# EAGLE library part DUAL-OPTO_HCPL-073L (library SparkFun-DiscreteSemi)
HCPL-073L These high gain series couplers use a Light Emitting Diode and an integrated high gain photodetector to provide extremely high current transfer ratio between input and output. Separate pins for the photodiode and output stage result in LVTTL compatible saturation voltages and high speed operation. Where desired, the VCC and VO terminals may be tied together to achieve conventional photo-darlington operation. A base access terminal allows a gain bandwidth adjustment to be made. These optocouplers are for use in LVTTL/LVCMOS or other low power applications. A 400% minimum current transfer ratio is guaranteed over 0 to +70˚C operating range for only 0.5 mA of LED current. Digikey Link
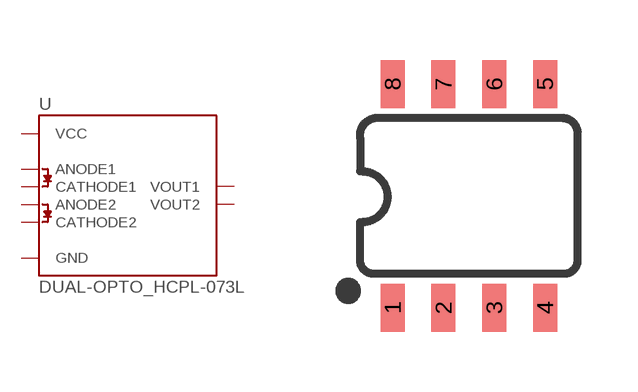
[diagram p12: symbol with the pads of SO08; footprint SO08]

Designator prefix U

## DUAL-OPTO_HCPL-073LSOIC-8 (PROD_ID: IC-15070)  [SO08]
1  ANODE1  in
2  CATHODE1  in
3  CATHODE2  in
4  ANODE2  in
5  GND  pwr
6  VOUT2  out
7  VOUT1  out
8  VCC  pwr

## Footprint SO08 (pad centres in mm)
SOIC, 0.15 inch width
smd 0.6 x 1.2: 1 -1.905,-2.8; 2 -0.635,-2.8; 3 0.635,-2.8; 4 1.905,-2.8; 5 1.905,2.8; 6 0.635,2.8; 7 -0.635,2.8; 8 -1.905,2.8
